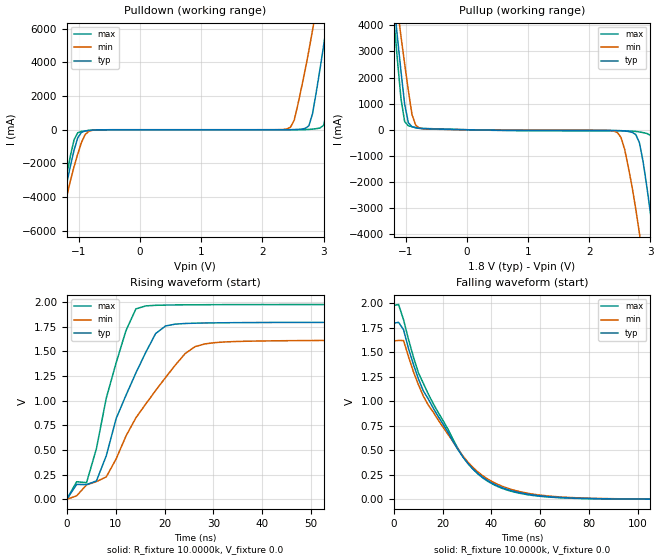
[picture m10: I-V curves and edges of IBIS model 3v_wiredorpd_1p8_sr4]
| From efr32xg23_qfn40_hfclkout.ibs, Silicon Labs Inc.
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|   Model 3v_wiredorpd_1p8_sr4
[Model]  3v_wiredorpd_1p8_sr4
Model_type Output
Polarity   Non-Inverting
Enable   Active-Low
C_comp   1.6300pF   1.4000pF   2.7000pF
[Temperature Range]   25.0000   0.1250k   -40.0000
[Pullup Reference]   1.8000V   1.6200V   1.9800V
[Pulldown Reference]   0.0V   0.0V   0.0V
[POWER Clamp Reference]   1.8000V   1.6200V   1.9800V
[GND Clamp Reference]   0.0V   0.0V   0.0V
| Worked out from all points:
|   slope of the pulldown table from 0 to 0.27 V, typ, clamps not added: 44.9 kohm
|   slope of the pullup table from 0 to 0.27 V, typ, clamps not added: 26.3 ohm
|   rising waveform, R_fixture 10.0000k, V_fixture 0.0: 20-80 % time 8.2ns typ, 11.9ns min, 5.94ns max; typ from 0 V to 1.8 V
|   falling waveform, R_fixture 10.0000k, V_fixture 0.0: 20-80 % time 23.3ns typ, 24.3ns min, 22.9ns max; typ from 1.8 V to 0.001 V
[Pulldown]
|Voltage   I(typ)   I(min)   I(max)
-1.8V     -14.24A    -14.11A    -14.46A
-1.38V    -6.468A    -6.98A     -6.16A
-1.14V    -2.14A     -3.023A    -1.532A
-1.02V    -472.4mA   -1.439A    -175.3mA
-780mV    -21.14mA   -32.29mA   -22.9mA
2.46V     4.055mA    156.9mA    301.8uA
2.76V     235.9mA    4.702A     17.88mA
2.82V     958.6mA    5.911A     36.7mA
2.94V     3.56A      8.545A     100.9mA
3.06V     6.47A      11.36A     1.157A
3.24V     11.25A     15.63A     5.98A
3.6V      20.85A     23.6A      16.79A
[Pullup]
|Voltage   I(typ)   I(min)   I(max)
-1.8V     20.86A     19.71A     22.08A
-1.2V     4.996A     5.919A     4.326A
-1.08V    2.239A     3.576A     1.188A
-960mV    270.1mA    1.509A     153.5mA
-840mV    73.79mA    176mA      86.18mA
-720mV    40.46mA    33.96mA    52.78mA
2.46V     -30.6mA    -110.1mA   -41.67mA
2.58V     -47.09mA   -768.5mA   -43.99mA
2.82V     -498.4mA   -3.974A    -84.68mA
3V        -3.194A    -6.995A    -216.9mA
3.24V     -7.63A     -11.15A    -3.824A
3.6V      -14.27A    -16.88A    -11.03A
[Ramp]
| variable   typ   min   max
dV/dt_r  1.0775/8.2038n   0.9686/11.9490n   1.1861/5.9398n
dV/dt_f  0.1964/25.9671n   0.1553/27.6999n   0.2452/24.5618n
R_load = 10.0000k
[Rising Waveform]
R_fixture= 10.0000k
V_fixture= 0.0
V_fixture_min= 0.0
V_fixture_max= 0.0
|time   V(typ)   V(min)   V(max)
0s        4.6uV      60.57uV    4.524uV
4.04ns    149.4mV    146.7mV    169mV
6.061ns   186.6mV    179.6mV    513.8mV
8.081ns   442.3mV    227.8mV    1.028V
12.12ns   1.057V     643.6mV    1.714V
16.16ns   1.492V     967.7mV    1.963V
20.2ns    1.759V     1.236V     1.971V
24.24ns   1.784V     1.48V      1.973V
30.3ns    1.79V      1.59V      1.975V
200ns     1.796V     1.614V     1.977V
[Falling Waveform]
R_fixture= 10.0000k
V_fixture= 0.0
V_fixture_min= 0.0
V_fixture_max= 0.0
|time   V(typ)   V(min)   V(max)
0s        1.796V     1.614V     1.977V
2.02ns    1.804V     1.62V      1.986V
4.04ns    1.73V      1.619V     1.831V
10.1ns    1.231V     1.17V      1.292V
14.14ns   1.025V     961.6mV    1.075V
26.26ns   508.2mV    513.5mV    519.8mV
34.34ns   266.2mV    282.3mV    262.2mV
44.44ns   119mV      133.1mV    112mV
76.77ns   10.96mV    14.4mV     8.932mV
200ns     728.3uV    1.014mV    567.9uV
